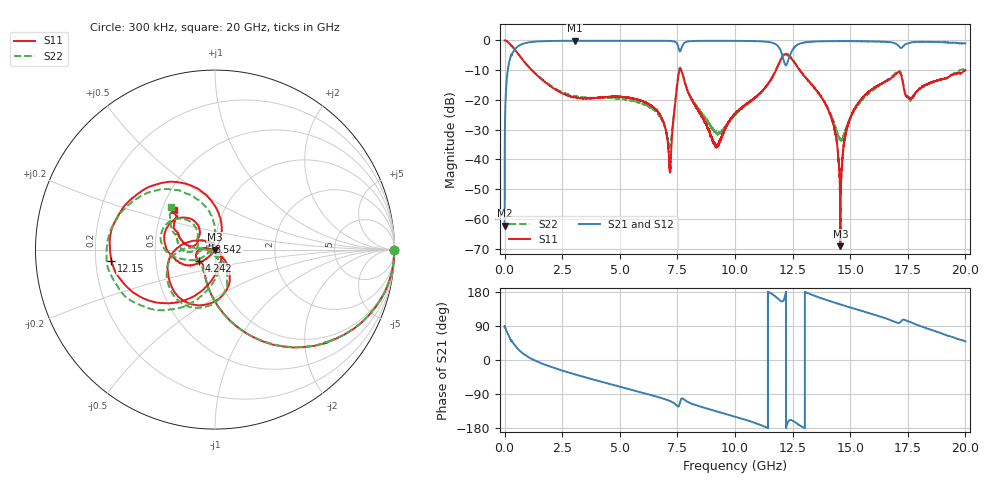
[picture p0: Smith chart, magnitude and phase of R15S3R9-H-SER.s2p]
!{R15S3R9}
!Johanson Technology Inc.
!www.johansontechnology.com
!Test Board Conditions:
!Substrate Type  RO4350B
!Substrate Thickness  20 mil
!Substrate Dk  3.66
!TL Type: GCPW
!TL Trace Width  34 mil
!TL Gap  10 mil
!Electrode orientation  Horizontal
!DUT TOPOLOGY	SERIES
!Mounting Pad LxW  26x52 mil
! Created Sat Feb  6 13:55:52 2021
# hz S ma R 50
! 2 Port Network Data from SP1.SP block
! freq  magS11  angS11  magS21  angS21  magS12  angS12  magS22  angS22
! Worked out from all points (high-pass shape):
!   20001 points, 300 kHz to 20 GHz, reference 50 ohm
!   highest |S21| = -0.10 dB at 3.043 GHz (marker M1); lowest = -62.3 dB at 300 kHz (marker M2)
!   |S21| within 3 dB of the highest: 435.1 MHz to 7.573 GHz (7.138 GHz wide, 178 % of centre); 12.51 GHz to end of sweep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
!   lowest |S11| = -69.1 dB at 14.57 GHz (marker M3), VSWR 1.00, Z = 50 + j0.0333 ohm
!   |S11| at or under -10 dB: 1.182 GHz to 7.584 GHz (6.402 GHz wide, 146 % of centre); 7.659 GHz to 11.78 GHz (4.12 GHz wide, 42.4 % of centre); 12.81 GHz to 19.99 GHz (7.173 GHz wide, 43.7 % of centre)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
!   |S22| runs from -35.8 to 0.0 dB; largest |S21 - S12| = 0.015
!   S11 on the Smith chart (normalised r, x): 300 kHz: open; 4.242 GHz: 0.83, -0.11; 8.542 GHz: 0.93, +0.08; 12.15 GHz: 0.27, -0.05; 20 GHz: 0.58, +0.28
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300000  1 -0.2  0.0007679 86.0  0.000745 83.7  0.9982 -0.2
1.163e8  0.9609 -17.6  0.2722 72.2  0.2729 72.2  0.9602 -17.4
3.513e8  0.78 -43.1  0.6186 46.6  0.6207 46.6  0.7797 -42.9
1.1703e9  0.3196 -86.5  0.9417 3.1  0.9393 3.1  0.3239 -86.3
3.0433e9  0.1103 -126.4  0.9885 -37.7  0.9874 -37.7  0.1158 -130.0
3.3343e9  0.107 -131.0  0.9882 -42.8  0.9874 -42.8  0.1113 -135.8
4.2423e9  0.1104 -145.1  0.9869 -58.0  0.9858 -58.0  0.1085 -152.2
6.6673e9  0.06219 171.6  0.9864 -97.8  0.9872 -97.8  0.05826 -179.5
7.1763e9  0.006005 -122.4  0.9813 -108.2  0.9803 -108.2  0.01689 -114.3
7.6393e9  0.3295 -131.6  0.6776 -105.8  0.6795 -105.8  0.3448 -131.3
8.5423e9  0.05386 127.6  0.9835 -123.7  0.9845 -123.7  0.06086 179.3
9.2043e9  0.01652 31.3  0.9873 -135.5  0.9867 -135.5  0.02755 -129.9
1.00003e10  0.0587 -53.8  0.9839 -149.5  0.9842 -149.4  0.05631 -71.5
1.15343e10  0.2125 -103.5  0.9302 176.6  0.9305 176.8  0.2155 -98.5
1.21453e10  0.5801 -173.7  0.4179 162.9  0.4224 162.4  0.5936 -165.3
1.33343e10  0.181 80.6  0.9519 172.1  0.9511 172.1  0.181 95.4
1.42113e10  0.04621 60.5  0.9735 153.6  0.9737 153.6  0.05073 94.6
1.45723e10  0.0003489 72.4  0.9787 146.7  0.9754 146.7  0.02143 147.4
1.50943e10  0.06056 -132.3  0.9743 136.8  0.9735 137.2  0.05844 -149.2
1.66673e10  0.2177 -163.3  0.9409 107.0  0.9301 107.0  0.2245 -168.8
1.76233e10  0.1051 158.7  0.9179 100.0  0.9182 99.7  0.09778 168.5
2e10  0.317 136.0  0.8922 49.0  0.8842 48.7  0.3404 135.6
